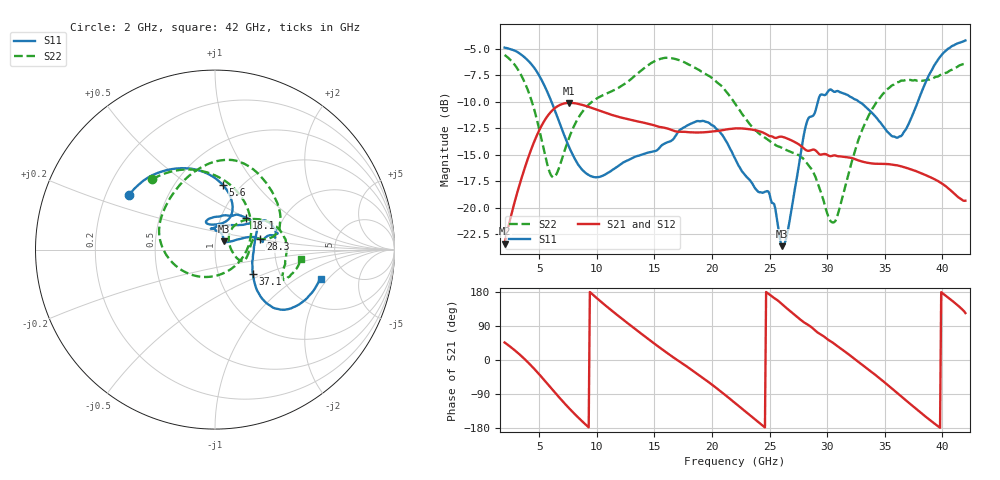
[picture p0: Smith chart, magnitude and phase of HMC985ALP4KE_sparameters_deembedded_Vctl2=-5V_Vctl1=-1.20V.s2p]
!s2p File: Measurements: S11, S21, S12, S22
# GHz S dB R 50.0
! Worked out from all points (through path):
!   401 points, 2 GHz to 42 GHz, reference 50 ohm
!   highest |S21| = -10.12 dB at 7.6 GHz (marker M1); lowest = -23.4 dB at 2 GHz (marker M2)
!   lowest |S11| = -23.6 dB at 26.1 GHz (marker M3), VSWR 1.14, Z = 54.8 + j4.97 ohm
!   |S11| at or under -10 dB: 6.066 GHz to 29.19 GHz (23.12 GHz wide, 131 % of centre); 32.75 GHz to 37.87 GHz (5.124 GHz wide, 14.5 % of centre)
!   |S22| runs from -21.4 to -5.6 dB; largest |S21 - S12| = 0.00031
!   S11 on the Smith chart (normalised r, x): 2 GHz: 0.30, +0.26; 5.6 GHz: 0.83, +0.69; 18.1 GHz: 1.31, +0.50; 28.3 GHz: 1.66, +0.20; 37.1 GHz: 1.46, -0.42; 42 GHz: 3.20, -1.71
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2  -4.91 147.9  -23.37 46.2  -23.37 46.2  -5.60 131.6
3.6  -5.71 121.4  -16.75 6.4  -16.75 6.4  -7.86 87.1
4.7  -7.02 100.4  -13.43 -27.5  -13.43 -27.5  -11.26 45.2
5.6  -8.82 82.9  -11.55 -58.6  -11.56 -58.6  -15.45 -7.6
6.4  -10.93 70.7  -10.57 -86.9  -10.58 -86.9  -17.01 -75.7
7.6  -14.28 65.2  -10.12 -127.4  -10.12 -127.4  -13.40 -146.2
8.7  -16.38 75.2  -10.29 -160.9  -10.30 -160.9  -11.03 -177.2
12  -15.96 108.3  -11.47 113.3  -11.47 113.3  -8.62 136.0
15.4  -14.40 79.6  -12.37 34.3  -12.38 34.4  -6.02 85.2
18.1  -12.11 45.9  -12.88 -23.2  -12.89 -23.1  -6.56 52.9
20  -12.22 36.7  -12.81 -65.0  -12.82 -65.0  -7.76 27.0
22  -15.34 53.0  -12.53 -113.5  -12.53 -113.5  -10.18 11.7
24.9  -18.46 95.7  -13.19 174.8  -13.20 174.9  -13.63 10.9
26.1  -23.61 43.2  -13.31 146.9  -13.32 146.9  -14.38 -2.0
28.3  -11.74 12.7  -14.63 93.4  -14.63 93.5  -15.87 -22.9
28.7  -11.38 9.3  -14.53 85.0  -14.54 85.0  -16.44 -23.1
30.6  -9.07 15.9  -15.06 43.1  -15.06 43.1  -21.36 21.2
33.1  -10.25 31.5  -15.66 -13.9  -15.67 -13.9  -12.50 44.3
35.4  -13.01 9.0  -15.90 -69.6  -15.90 -69.5  -8.69 19.6
37.1  -12.03 -32.7  -16.32 -113.1  -16.32 -113.1  -7.97 0.0
39.7  -5.93 -41.6  -17.53 -176.6  -17.53 -176.5  -7.58 -23.8
42  -4.24 -15.7  -19.33 123.8  -19.33 123.8  -6.35 -6.0
